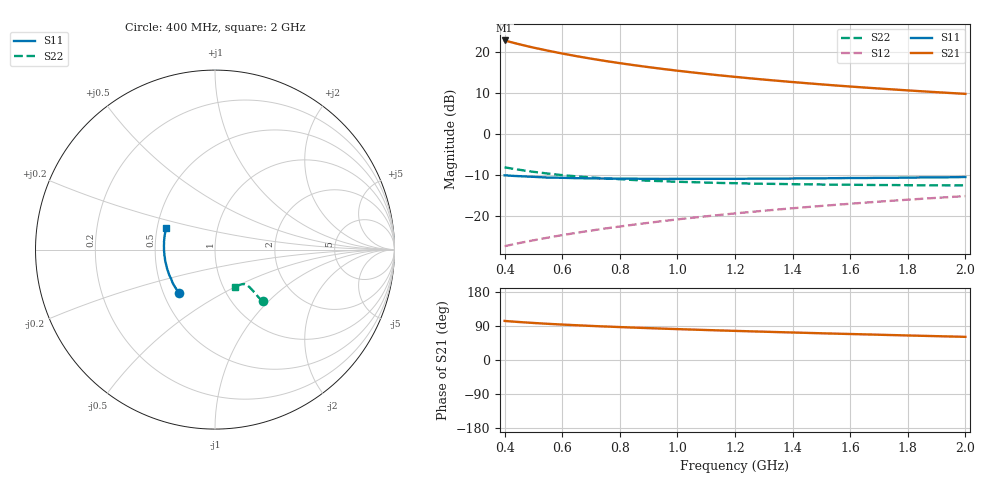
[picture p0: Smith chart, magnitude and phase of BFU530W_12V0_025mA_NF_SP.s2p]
! Filename:  P:\Prog\Test\Noise\ATS_data\Testdata_Net\06 Compressed Noise after Statistics\BFU530W_APM2013_09_A05_12p0V_025mA_NF_CM01_D.sf
! Date/Time: Tue 26/Mar/2013 18:06:01
! BFU530W_APM2013_09_A05_12p0V_1to25mA_NF_CM01_Bias9_R.sf
! Noise Parameter Data File
! BFU530W_APM2013_09_A05_12p0V_1to25mA_NF_CM01
! Date/time: Thu Mar 21 22:54:15 2013
! VAR V_out= 12.000000
! VAR I_out= 25.000000
! VAR V_in= 0.758200
! VAR I_in= 0.231450
! Device data file deembeded for feedlines and parallel
! Original file: \06 Compressed Noise after Statistics\BFU530W_APM2013_09_A05_12p0V_025mA_NF_CM01_R.sf
! Feed-files: PR019V01_070313_Feed1.s2p, PR019V01_070313_Feed2.s2p
! Parallel-file: PR019V01_070313_Par.s2p
# MHz S MA R 50
!  Freq-MHz  S11-mag  S11-arg  S21-mag  S21-arg  S12-mag  S12-arg  S22-mag  S22-arg
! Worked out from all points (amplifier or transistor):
!   37 points, 400 MHz to 2 GHz, reference 50 ohm
!   highest |S21| = 22.8 dB at 400 MHz (marker M1)
!   |S21| within 3 dB of that: start of sweep to 586.9 MHz
!   unconditionally stable (mu >= 1): 1.07 GHz to end of sweep
!   at 500 MHz: K = 0.88, MSG = 23.5 dB, |S12| = -25.9 dB
!   at 1.1 GHz: K = 1.00, MAG = 17.1 dB, |S12| = -20.1 dB
!   at 2 GHz: K = 1.01, MAG = 11.9 dB, |S12| = -15.1 dB
!   lowest NFmin = 1.20 dB at 440 MHz
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400  0.3134 -130.0  13.77 103.1  0.04291 66.4  0.3922 -47.3
420  0.3101 -132.7  13.19 101.9  0.04441 66.7  0.3812 -47.5
433  0.3078 -134.4  12.84 101.2  0.04541 66.9  0.3743 -47.5
460  0.3047 -137.3  12.16 99.8  0.04748 67.3  0.3621 -47.6
500  0.3002 -141.7  11.27 97.8  0.05055 67.8  0.3454 -47.5
550  0.2938 -146.3  10.34 95.5  0.05452 68.5  0.3292 -47.4
600  0.2922 -150.4  9.546 93.5  0.05847 68.9  0.3149 -47.3
650  0.289 -154.1  8.859 91.7  0.06241 69.2  0.3043 -47.3
700  0.2876 -157.6  8.263 90.0  0.06643 69.6  0.295 -47.4
750  0.2861 -160.6  7.742 88.4  0.07045 69.9  0.2867 -47.3
800  0.2846 -163.6  7.284 86.9  0.07451 70.1  0.2809 -47.6
850  0.2848 -166.3  6.878 85.5  0.07856 70.3  0.2743 -47.7
950  0.2831 -171.0  6.189 82.8  0.0868 70.5  0.2655 -48.1
1050  0.2834 -175.2  5.629 80.3  0.09505 70.6  0.2587 -48.7
1150  0.2844 -179.3  5.161 78.0  0.1033 70.5  0.2527 -49.5
1200  0.284 178.9  4.96 76.8  0.1076 70.4  0.2512 -50.1
1250  0.2847 177.1  4.769 75.7  0.1116 70.3  0.2486 -50.5
1350  0.2855 173.9  4.438 73.6  0.1201 70.0  0.2459 -51.7
1500  0.2878 169.3  4.017 70.5  0.1327 69.5  0.2421 -53.8
1650  0.2904 165.0  3.675 67.6  0.1453 68.8  0.2393 -55.9
1750  0.2923 162.5  3.483 65.7  0.1538 68.3  0.2384 -57.3
2000  0.2987 156.4  3.079 61.1  0.1749 66.9  0.2364 -61.8
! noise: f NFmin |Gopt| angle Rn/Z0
400  1.207  0.2256  -174  0.0961
460  1.202  0.2276  -174.2  0.0996
600  1.226  0.2374  -170.1  0.0947
800  1.271  0.2478  -166.5  0.0936
1000  1.274  0.2586  -162.3  0.0962
1200  1.266  0.2685  -160  0.1004
1400  1.335  0.2715  -154.7  0.103
1600  1.35  0.2877  -151  0.1025
1800  1.376  0.2941  -147.6  0.1087
2000  1.409  0.3056  -144.4  0.1123
